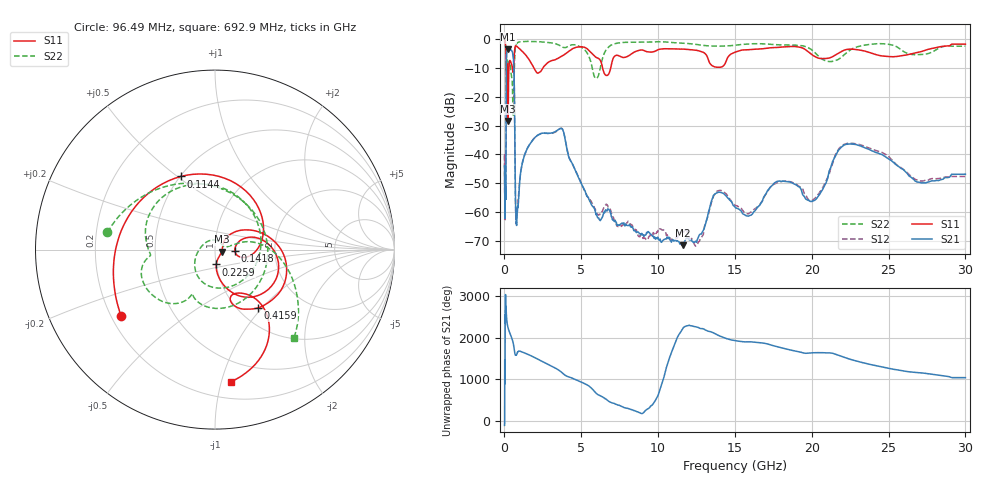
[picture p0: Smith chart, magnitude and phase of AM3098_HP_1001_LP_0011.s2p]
! Date/Time: Thu, Feb 28, 2019 8:40 AM
! Network Analyzer: Agilent Technologies E8364B Rev: A.07.50.67
! Sweep from 0.010 to 30.000 GHz, 1601 Points, Sweep Type: LOG
! Power Supply: 5.023 V, 0.002 A
# Hz S DB R 50
!freq MagS11 AngS11 MagS21 AngS21 MagS12 AngS12 MagS22 AngS22
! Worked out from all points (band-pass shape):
!   1601 points, 10 MHz to 30 GHz, reference 50 ohm
!   highest |S21| = -3.36 dB at 238.7 MHz (marker M1); lowest = -71.7 dB at 11.59 GHz (marker M2)
!   |S21| within 3 dB of the highest: 129.4 MHz to 580.5 MHz (451 MHz wide, 127 % of centre)
!   lowest |S11| = -28.3 dB at 237.5 MHz (marker M3), VSWR 1.08, Z = 53.8 - j1.28 ohm
!   |S11| at or under -10 dB: 198.6 MHz to 289.6 MHz (91.02 MHz wide, 37.3 % of centre); 1.918 GHz to 2.494 GHz (575.2 MHz wide, 26.1 % of centre); 6.39 GHz to 6.911 GHz (521.2 MHz wide, 7.84 % of centre)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
!   |S22| runs from -26.3 to -0.5 dB; largest |S21 - S12| = 0.016
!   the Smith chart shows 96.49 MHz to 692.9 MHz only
!   S11 on the Smith chart (normalised r, x): 96.49 MHz: 0.24, -0.30; 114.4 MHz: 0.50, +0.51; 141.8 MHz: 1.25, -0.02; 225.9 MHz: 1.00, -0.17; 415.9 MHz: 1.22, -0.95; 692.9 MHz: 0.33, -1.07
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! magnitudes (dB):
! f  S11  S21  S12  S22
! 10 MHz  -0.3  -44.1  -40.2  -0.5
! 38.04 MHz  -0.5  -59.8  -59.0  -0.8
! 96.49 MHz  -3.9  -44.2  -43.6  -4.3
! 114.4 MHz  -6.9  -16.7  -16.7  -10.6
! 141.8 MHz  -19.1  -4.7  -4.6  -11.0
! 144.7 MHz  -18.9  -4.5  -4.5  -10.7
! 184.9 MHz  -8.6  -4.0  -3.9  -7.1
! 225.9 MHz  -21.6  -3.4  -3.4  -8.8
! 237.5 MHz  -28.3  -3.4  -3.3  -8.9
! 238.7 MHz  -28.3  -3.4  -3.3  -8.9
! 415.9 MHz  -7.9  -3.7  -3.6  -11.1
! 550.5 MHz  -11.4  -5.1  -5.1  -24.2
! 630.1 MHz  -6.1  -12.9  -12.9  -13.6
! 692.9 MHz  -2.6  -44.6  -45.1  -3.6
! 781.4 MHz  -2.3  -64.4  -63.8  -1.5
! 2.084 GHz  -11.4  -33.7  -33.6  -0.7
! 3.723 GHz  -5.8  -31.0  -30.9  -2.4
! 7.926 GHz  -6.1  -64.6  -64.1  -1.0
! 11.59 GHz  -3.4  -71.7  -67.1  -1.3
! 20.2 GHz  -5.9  -56.0  -55.3  -4.6
! 22.56 GHz  -3.4  -36.4  -36.1  -3.5
! 30 GHz  -1.6  -46.9  -47.7  -2.3
